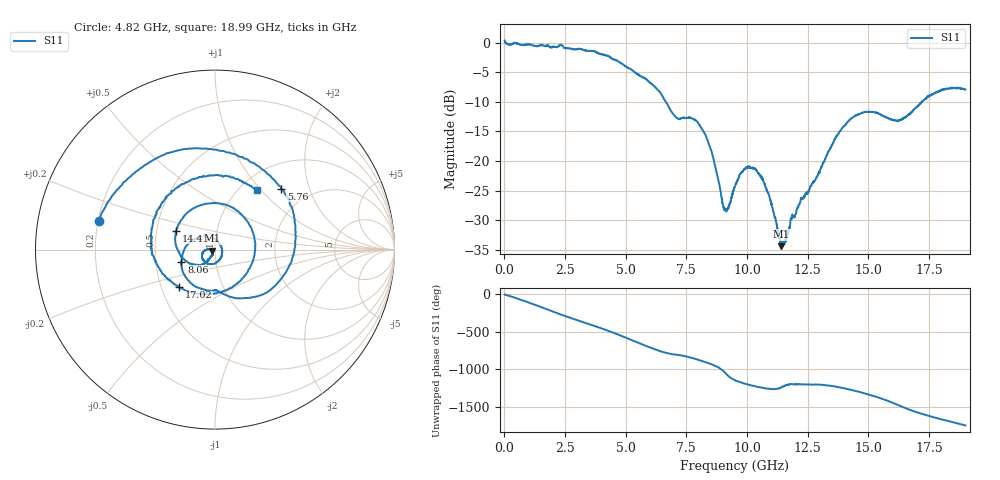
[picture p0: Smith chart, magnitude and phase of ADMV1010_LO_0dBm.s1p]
! Analog Devices, Inc.
! 1 Analog Way
! Wilmington, MA 01887
! http://www.analog.com
! Date:  2021-09-07 NN
! Board Name:  ADMV1010-EVALZ Revision B with ADMV1010AEZ installed
! File Description:  S-Parameters for evaluation board without connectors or board loss de-embedded
! File Generation:  Calibrated Network Analyzer
! Chip Part Number:  ADMV1010
! Chip Description:  GaAs, MMIC, IQ Downconverter
! Chip Frequency:  12.6 to 15.4 GHz
! Chip Package:  LCC, 4.9 x 4.9 x 1 mm
! Chip State:
!  Temperature:  25C
!  LO Power:  0dBm
! Note:
!  Analog Devices supplies this data as a sample of measured data at the evaluation board
!  ports for this product.  Your particular data for this product may vary.
!  Analog Devices reserves the right to change this data at anytime.
!  All lines below in this file are as is from the Network Analyzer.
!Keysight Technologies,N5245A,MY49151104,A.10.65.16
!Date: Wednesday, August 25, 2021 14:18:15
!Correction: S11(Full 2 Port(1,2))
!S1P File: Measurement: S11:
# Hz S  dB  R 50
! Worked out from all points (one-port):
!   1900 points, 10 MHz to 19 GHz, reference 50 ohm
!   lowest |S11| = -34.4 dB at 11.4 GHz (marker M1), VSWR 1.04, Z = 48.2 - j0.618 ohm
!   |S11| at or under -10 dB: 6.644 GHz to 17.21 GHz (10.56 GHz wide, 88.6 % of centre)
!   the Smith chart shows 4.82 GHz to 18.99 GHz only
!   S11 on the Smith chart (normalised r, x): 4.82 GHz: 0.20, +0.12; 5.76 GHz: 1.46, +1.33; 8.06 GHz: 0.68, -0.09; 14.45 GHz: 0.63, +0.14; 17.02 GHz: 0.62, -0.28; 18.99 GHz: 1.20, +0.95
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1e7  0.36 -3.8
8.4e8  -0.39 -91.0
1.51e9  -0.36 -170.5
1.86e9  -0.76 147.2
2.39e9  -0.54 83.7
3.1e9  -1.04 4.7
3.8e9  -1.63 -72.2
4.22e9  -2.17 -119.5
4.76e9  -3.38 173.9
4.82e9  -3.51 166.2
5.27e9  -4.64 106.9
5.76e9  -5.98 42.6
6.43e9  -8.48 -38.5
7.14e9  -12.84 -87.4
8.06e9  -14.02 -160.4
9.07e9  -28.29 43.3
9.51e9  -24.15 -66.9
1.04e10  -21.71 -151.4
1.14e10  -34.38 -160.4
1.188e10  -29.43 -116.7
1.426e10  -12.94 168.9
1.445e10  -12.38 153.9
1.584e10  -12.82 16.4
1.663e10  -12.22 -88.6
1.702e10  -10.81 -133.6
1.783e10  -8.31 150.1
1.899e10  -7.88 54.9
1.9e10  -7.96 53.0
